FUNCTION_BLOCK AxisModule
VAR
	applicationState : I_ApplicationState;
	moduleInitSubstate : I_Substate;
	moduleAxisPowerSubstate : I_Substate;
END_VAR

METHOD PUBLIC Execute
VAR_INPUT
END_VAR
IF applicationState.CurrentState.IsEqual(moduleInitSubstate) THEN
	// do what I do to init,
	applicationState.MoveNext();
	
ELSIF applicationState.CurrentState.IsEqual(moduleAxisPowerSubstate) THEN
	// do what I do to power on,
	applicationState.MoveNext();
END_IF
END_METHOD

METHOD FB_init : BOOL
VAR_INPUT
	bInitRetains : BOOL; // if TRUE, the retain variables are initialized (warm start / cold start)
	bInCopyCode : BOOL;  // if TRUE, the instance afterwards gets moved into the copy code (online change)
	ApplicationState : I_ApplicationState;
	InitSubstate : I_Substate;
	AxisPowerSubstate : I_Substate;
END_VAR
THIS^.applicationState := ApplicationState;
moduleInitSubstate := InitSubstate;
moduleAxisPowerSubstate := AxisPowerSubstate;
END_METHOD

END_FUNCTION_BLOCK
